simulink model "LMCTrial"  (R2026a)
settings: Solver=ode1  StopTime=0.4  FixedStep=0.00001
libraries: LoomingNeuronLibrary x11

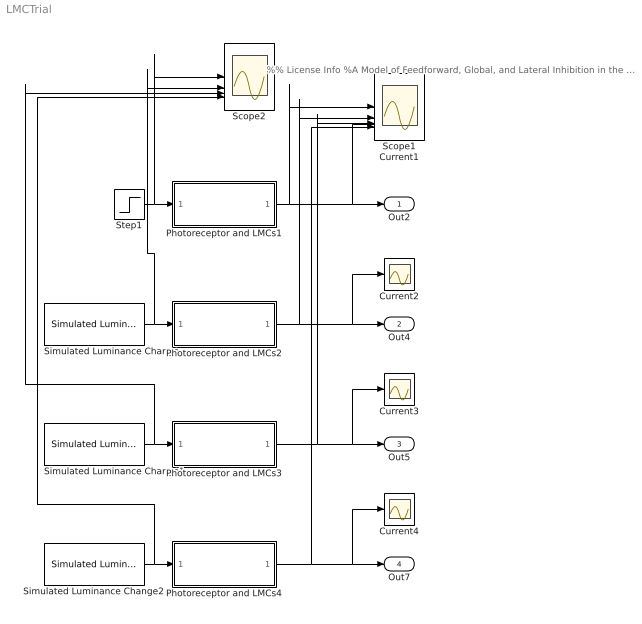
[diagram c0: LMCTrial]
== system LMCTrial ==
  note: %% License Info %A Model of Feedforward, Global, and Lateral Inhibition in the Locust Visual System. %This model examines the architecture and function of inhibitory mechanisms in the %visual system of locusts, namely those involved in the processing of inputs to a %key looming-sensitive neuron, the lobula giant movement detector (LGMD). %Copyright (c) 2026, Erik Olson, Travis Wiens, and Jack Gray %CITATION: %When using the model code for scientific publications, cite the following work: %Olson EGN, Wiens TK, Gray JR. A model of feedforward, global, and lateral inhibition %in the locust visual system predicts responses to looming stimuli. Biol Cybern. 2021 %Jun;115(3):245-265. doi: 10.1007/s00422-021-00876-8. Epub 2021 May 16. PMID: 33997912. %This program is free software: you can redistribute it and/or modify %it under the terms of the GNU General Public License as published by %the Free Software Foundation, either version 3 of the License, or %(at your option) any later version. %This program is distributed in the hope that it will be useful, %but WITHOUT ANY WARRANTY; without even the implied warranty of %MERCHANTABILITY or FITNESS FOR A PARTICULAR PURPOSE. See the %GNU General Public License for more details. %You should have received a copy of the GNU General Public License %along with this program. If not, see <https://www.gnu.org/licenses/>. %Contact: erik.olson@usask.ca
  Current{1..4} (4 alike) : Scope
  Photoreceptor and LMCs1 : Subsystem
  Photoreceptor and LMCs2 : Subsystem
  Photoreceptor and LMCs3 : Subsystem
  Photoreceptor and LMCs4 : Subsystem
  Scope1 : Scope  NumInputPorts=4
  Scope2 : Scope  NumInputPorts=4
  Simulated Luminance Change : LoomingNeuronLibrary/Simulated Luminance Change  duration=0.083  start=0
  Simulated Luminance Change1 : LoomingNeuronLibrary/Simulated Luminance Change  duration=0.183  start=0
  Simulated Luminance Change2 : LoomingNeuronLibrary/Simulated Luminance Change  duration=0.350  start=0
  Step1 : Step  Time=0.00001  InitialValue=1  FinalValue=0  SampleTime=0
  Out2 : Outport  VectorParamsAs1DForOutWhenUnconnected=off
  Out4 : Outport  Port=2  VectorParamsAs1DForOutWhenUnconnected=off
  Out5 : Outport  Port=3  VectorParamsAs1DForOutWhenUnconnected=off
  Out7 : Outport  Port=4  VectorParamsAs1DForOutWhenUnconnected=off
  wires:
  Simulated Luminance Change/1 -> Scope2/2, Photoreceptor and LMCs2/1(In1)
  Simulated Luminance Change1/1 -> Scope2/3, Photoreceptor and LMCs3/1(In1)
  Photoreceptor and LMCs4/1(Out1) -> Out7/1, Current4/1, Scope1/4
  Step1/1 -> Scope2/1, Photoreceptor and LMCs1/1(In1)
  Photoreceptor and LMCs3/1(Out1) -> Out5/1, Current3/1, Scope1/3
  Photoreceptor and LMCs1/1(Out1) -> Out2/1, Current1/1, Scope1/1
  Photoreceptor and LMCs2/1(Out1) -> Out4/1, Current2/1, Scope1/2
  Simulated Luminance Change2/1 -> Scope2/4, Photoreceptor and LMCs4/1(In1)

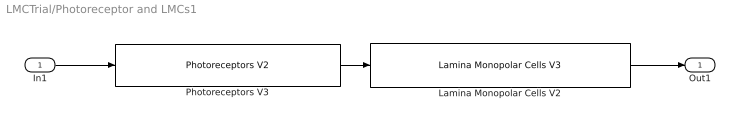
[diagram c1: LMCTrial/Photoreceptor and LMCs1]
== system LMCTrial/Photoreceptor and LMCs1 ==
  In1 : Inport
  Lamina Monopolar Cells V2 : LoomingNeuronLibrary/Lamina Monopolar Cells V3  K_LMC=K_LMC  gamma_1=b
  Photoreceptors V3 : LoomingNeuronLibrary/Photoreceptors V2  K_photoD=K_photoD  K_photoP=K_photoP  alpha_1=a_1  alpha_2=a_2
  Out1 : Outport  VectorParamsAs1DForOutWhenUnconnected=off
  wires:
  Lamina Monopolar Cells V2/1 -> Out1/1
  Photoreceptors V3/1 -> Lamina Monopolar Cells V2/1
  In1/1 -> Photoreceptors V3/1

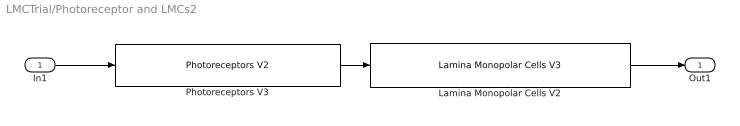
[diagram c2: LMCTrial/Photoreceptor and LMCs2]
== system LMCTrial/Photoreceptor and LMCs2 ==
  In1 : Inport
  Lamina Monopolar Cells V2 : LoomingNeuronLibrary/Lamina Monopolar Cells V3  K_LMC=K_LMC  gamma_1=b
  Photoreceptors V3 : LoomingNeuronLibrary/Photoreceptors V2  K_photoD=K_photoD  K_photoP=K_photoP  alpha_1=a_1  alpha_2=a_2
  Out1 : Outport  VectorParamsAs1DForOutWhenUnconnected=off
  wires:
  Photoreceptors V3/1 -> Lamina Monopolar Cells V2/1
  Lamina Monopolar Cells V2/1 -> Out1/1
  In1/1 -> Photoreceptors V3/1

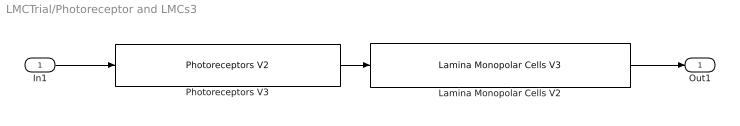
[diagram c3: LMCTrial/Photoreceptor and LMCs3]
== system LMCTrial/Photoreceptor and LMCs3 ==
  In1 : Inport
  Lamina Monopolar Cells V2 : LoomingNeuronLibrary/Lamina Monopolar Cells V3  K_LMC=K_LMC  gamma_1=b
  Photoreceptors V3 : LoomingNeuronLibrary/Photoreceptors V2  K_photoD=K_photoD  K_photoP=K_photoP  alpha_1=a_1  alpha_2=a_2
  Out1 : Outport  VectorParamsAs1DForOutWhenUnconnected=off
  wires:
  Photoreceptors V3/1 -> Lamina Monopolar Cells V2/1
  Lamina Monopolar Cells V2/1 -> Out1/1
  In1/1 -> Photoreceptors V3/1

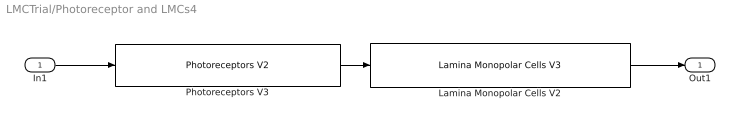
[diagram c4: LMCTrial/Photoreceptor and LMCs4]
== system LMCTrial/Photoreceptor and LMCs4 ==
  In1 : Inport
  Lamina Monopolar Cells V2 : LoomingNeuronLibrary/Lamina Monopolar Cells V3  K_LMC=K_LMC  gamma_1=b
  Photoreceptors V3 : LoomingNeuronLibrary/Photoreceptors V2  K_photoD=K_photoD  K_photoP=K_photoP  alpha_1=a_1  alpha_2=a_2
  Out1 : Outport  VectorParamsAs1DForOutWhenUnconnected=off
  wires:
  Photoreceptors V3/1 -> Lamina Monopolar Cells V2/1
  Lamina Monopolar Cells V2/1 -> Out1/1
  In1/1 -> Photoreceptors V3/1
